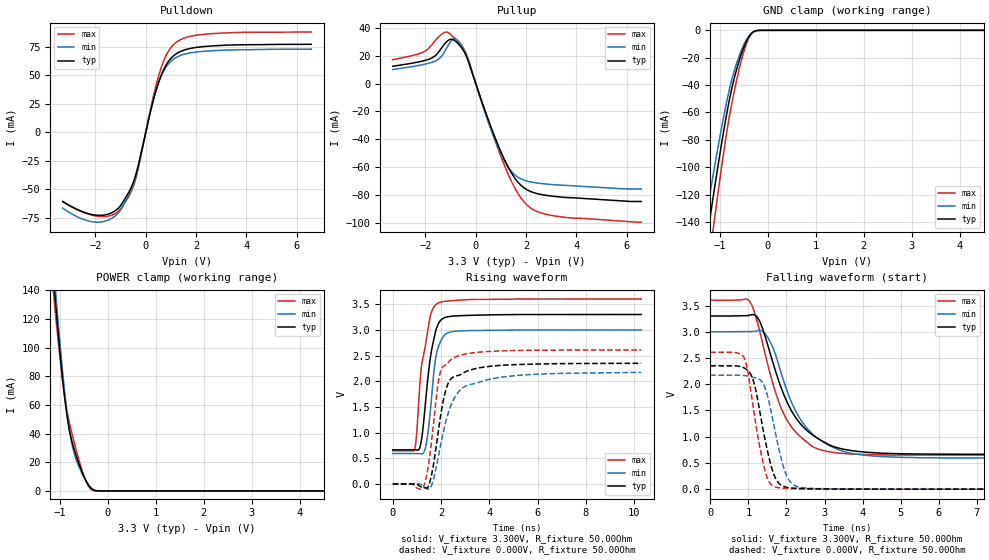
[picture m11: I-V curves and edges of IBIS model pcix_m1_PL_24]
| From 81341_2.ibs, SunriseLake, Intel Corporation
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[Model]   pcix_m1_PL_24
Model_type   I/O
Vinl = 1.155V
Vinh = 1.650V
Vmeas = 1.320V
Vref = 0.000V
Cref = 10.000pF
Rref = 25.000Ohm
|   typ   min   max
C_comp   7.500pF   6.000pF   9.000pF
[Voltage Range]   3.300V   3.000V   3.600V
[Temperature Range]   60.0   110.0   -5.0
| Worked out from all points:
|   slope of the pulldown table from 0 to 0.495 V, typ, clamps not added: 11.5 ohm
|   slope of the pullup table from 0 to 0.495 V, typ, clamps not added: 19.2 ohm
|   GND clamp passes 1 mA (typ) near -0.30 V on its own axis
|   POWER clamp passes 1 mA (typ) near -0.32 V on its own axis
|   falling waveform, V_fixture 3.300V, R_fixture 50.00Ohm: 20-80 % time 938ps typ, 920ps min, 785ps max; typ from 3.3 V to 0.664 V
|   rising waveform, V_fixture 3.300V, R_fixture 50.00Ohm: 20-80 % time 405ps typ, 327ps min, 428ps max; typ from 0.664 V to 3.3 V
|   rising waveform, V_fixture 0.000V, R_fixture 50.00Ohm: 20-80 % time 514ps typ, 792ps min, 399ps max; typ from 0 V to 2.35 V
|   falling waveform, V_fixture 0.000V, R_fixture 50.00Ohm: 20-80 % time 392ps typ, 399ps min, 361ps max; typ from 2.35 V to 0 V
[Pulldown]
|   Voltage   I(typ)   I(min)   I(max)
-3.3V     -60.68mA   -66.35mA   -60.38mA
-1.9V     -72.62mA   -78.65mA   -73.47mA
-1.35V    -70.33mA   -75.28mA   -72.48mA
-950mV    -62.47mA   -66.37mA   -65.34mA
-600mV    -49.2mA    -51.26mA   -52.88mA
-400mV    -37.34mA   -38.58mA   -40.7mA
200mV     19.46mA    19.83mA    21.55mA
500mV     43.22mA    42.9mA     48.76mA
850mV     60.55mA    58.59mA    69.21mA
1.25V     69.39mA    66.14mA    79.52mA
2.65V     75.76mA    71.55mA    86.51mA
6.575V    77.14mA    72.92mA    87.84mA
[GND Clamp]
|   Voltage   I(typ)   I(min)   I(max)
-3.3V     -632.5mA   -564.4mA   -725.5mA
-1.325V   -165.6mA   -144.4mA   -196mA
-1.3V     -159.5mA   -139mA     -189mA
-1.25V    -147.6mA   -128.4mA   -175.3mA
-1.2V     -135.8mA   -118mA     -161.6mA
-1.125V   -118.5mA   -102.6mA   -141.4mA
-850mV    -59.64mA   -50.8mA    -72.97mA
-650mV    -28.41mA   -23.93mA   -36.31mA
-450mV    -8.219mA   -7.112mA   -10.14mA
-350mV    -2.584mA   -2.413mA   -2.802mA
-250mV    -331.3uA   -398.2uA   -220.5uA
6.575V    0A         0A         0A
[Pullup]
|   Voltage   I(typ)   I(min)   I(max)
-3.3V     12.53mA    10.21mA    17.29mA
-1.8V     18.06mA    15.06mA    26.88mA
-1.4V     24.74mA    18.95mA    34.96mA
-1.1V     31.15mA    27.5mA     36.87mA
-850mV    31.18mA    32.3mA     33.03mA
-500mV    24.17mA    25.92mA    25.44mA
500mV     -26.06mA   -27.74mA   -27.36mA
1V        -49.11mA   -50.57mA   -52.5mA
1.5V      -66.72mA   -64.81mA   -73.41mA
2V        -76.02mA   -69.96mA   -86.8mA
3.2V      -81.34mA   -72.89mA   -95.43mA
6.575V    -84.85mA   -75.77mA   -99.75mA
[POWER Clamp]
|   Voltage   I(typ)   I(min)   I(max)
-3.3V     1.109A     1.089A     1.13A
-1.15V    154.7mA    163.7mA    144.9mA
-1.1V     134.6mA    143.1mA    126.5mA
-1.05V    115.4mA    123.1mA    109.5mA
-900mV    64.86mA    68.99mA    65.55mA
-800mV    41.99mA    41.86mA    47.4mA
-750mV    34.63mA    32.54mA    40.32mA
-650mV    23.51mA    20.95mA    27.23mA
-500mV    10.16mA    9.585mA    10.63mA
-400mV    3.792mA    4.116mA    3.102mA
-300mV    590.1uA    959uA      205.5uA
6.575V    0A         0A         0A
[Ramp]
R_load = 50.00Ohm
|   typ   min   max
dV/dt_r   1.410V/514.093ps   1.303V/790.185ps   1.564V/398.758ps
dV/dt_f   1.582V/936.718ps   1.445V/918.972ps   1.771V/784.893ps
[Falling Waveform]
V_fixture = 3.300V
V_fixture_min = 3.000V
V_fixture_max = 3.600V
R_fixture = 50.00Ohm
|   Time   V(typ)   V(min)   V(max)
0s        3.3V       3V         3.6V
1.04ns    3.316V     3.004V     3.573V
1.25ns    3.258V     3.022V     3.141V
1.46ns    2.864V     2.944V     2.52V
1.67ns    2.351V     2.649V     1.948V
1.91ns    1.84V      2.1V       1.464V
2.3ns     1.306V     1.41V      1.044V
2.79ns    981.6mV    985.4mV    776mV
4.25ns    695.7mV    633.2mV    656.9mV
10.3ns    663.8mV    592.2mV    648.3mV
[Rising Waveform]
V_fixture = 3.300V
V_fixture_min = 3.000V
V_fixture_max = 3.600V
R_fixture = 50.00Ohm
|   Time   V(typ)   V(min)   V(max)
0s        663.8mV    592.2mV    648.3mV
900ps     663.9mV    591.8mV    668.2mV
990ps     661.2mV    592mV      967.7mV
1.12ns    705.6mV    590.5mV    1.908V
1.2ns     886.5mV    585.8mV    2.315V
1.4ns     1.792V     807.5mV    2.83V
1.59ns    2.547V     1.576V     3.318V
1.85ns    3.076V     2.608V     3.514V
2.6ns     3.272V     2.975V     3.574V
10.3ns    3.3V       3V         3.6V
[Rising Waveform]
V_fixture = 0.000V
V_fixture_min = 0.000V
V_fixture_max = 0.000V
R_fixture = 50.00Ohm
|   Time   V(typ)   V(min)   V(max)
0s        633.1nV    3.572uV    45.54nV
1.28ns    -69.53mV   -47.29mV   -53.17mV
1.43ns    -74.8mV    -94.25mV   226.2mV
1.58ns    113.4mV    -60.47mV   715.9mV
1.95ns    1.22V      674.4mV    2.141V
2.23ns    1.873V     1.268V     2.328V
2.53ns    2.086V     1.65V      2.456V
3.03ns    2.187V     1.906V     2.531V
4.41ns    2.307V     2.072V     2.589V
10.3ns    2.35V      2.172V     2.607V
[Falling Waveform]
V_fixture = 0.000V
V_fixture_min = 0.000V
V_fixture_max = 0.000V
R_fixture = 50.00Ohm
|   Time   V(typ)   V(min)   V(max)
0s        2.35V      2.172V     2.607V
890ps     2.31V      2.165V     2.501V
980ps     2.264V     2.157V     2.264V
1.15ns    2.019V     2.126V     1.449V
1.42ns    1.009V     1.961V     399.7mV
1.54ns    608.9mV    1.67V      146.5mV
1.7ns     227.9mV    1.114V     43.56mV
2ns       35.25mV    262mV      14.86mV
2.36ns    12.73mV    35.84mV    6.244mV
10.3ns    633.1nV    3.572uV    45.54nV
